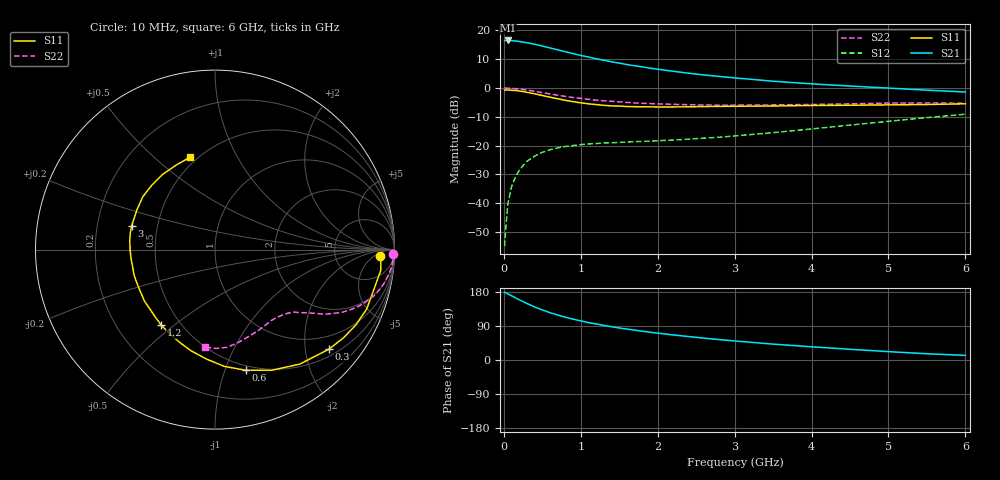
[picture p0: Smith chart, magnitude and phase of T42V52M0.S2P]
! Infineon Technologies  Discrete & RF Semiconductors
! BFR182T
! Si NPN RF Bipolar Junction Transistor in SC75
! VCE = 2.5 V  IC = 2 mA
! Common Emitter S-Parameters:  October  1999
# GHz  S  MA  R  50
!  f  S11  S21  S12  S22
! GHz  MAG  ANG  MAG  ANG  MAG  ANG  MAG  ANG
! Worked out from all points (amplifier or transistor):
!   36 points, 10 MHz to 6 GHz, reference 50 ohm
!   highest |S21| = 16.5 dB at 50 MHz (marker M1)
!   |S21| within 3 dB of that: start of sweep to 660.8 MHz
!   unconditionally stable (mu >= 1): 1.966 GHz to 4.331 GHz
!   at 250 MHz: K = 0.14, MSG = 21.5 dB, |S12| = -26.9 dB
!   at 1.4 GHz: K = 0.78, MSG = 14.0 dB, |S12| = -19.0 dB
!   at 6 GHz: K = 0.83, MSG = 3.9 dB, |S12| = -9.1 dB
!   lowest NFmin = 1.10 dB at 450 MHz
!   S11 on the Smith chart (normalised r, x): 10 MHz: 19, -9; 300 MHz: 0.66, -2.52; 600 MHz: 0.46, -1.18; 1.2 GHz: 0.39, -0.45; 3 GHz: 0.35, +0.12; 6 GHz: 0.46, +0.66
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0.01  0.9177 -2.4  6.671 178.4  0.0018 91.8  0.9899 -1.4
0.02  0.9257 -1.5  6.648 178.2  0.0029 92.8  0.9999 -1.2
0.05  0.9306 -7.2  6.704 174.7  0.0094 87.1  0.9939 -3.0
0.1  0.9132 -13.8  6.62 169.7  0.0194 80.7  0.988 -5.9
0.15  0.9077 -21.4  6.561 164.2  0.0284 77.4  0.9743 -8.7
0.25  0.8686 -34.4  6.297 154.1  0.045 71.1  0.9421 -13.8
0.3  0.8433 -41.1  6.118 149.2  0.0535 68.1  0.9233 -16.1
0.4  0.7937 -53.5  5.767 140.0  0.0659 61.9  0.8772 -20.3
0.5  0.7429 -64.8  5.357 132.2  0.0767 56.7  0.8321 -23.5
0.6  0.6937 -75.7  4.97 124.9  0.0848 52.7  0.7906 -26.2
0.8  0.6124 -94.3  4.275 112.9  0.0967 46.5  0.7162 -30.1
0.9  0.58 -103.1  3.958 107.8  0.1005 44.7  0.6849 -31.5
1.1  0.5326 -118.5  3.451 98.7  0.107 42.0  0.6375 -33.7
1.2  0.517 -125.3  3.225 95.1  0.1088 41.0  0.6171 -34.8
1.4  0.4908 -137.9  2.857 87.9  0.1125 40.0  0.5887 -36.7
1.6  0.4779 -149.8  2.561 81.5  0.1156 40.2  0.5629 -38.2
2.2  0.4703 -174.1  1.958 66.2  0.1254 43.9  0.5223 -44.4
3  0.483 163.9  1.501 50.3  0.1475 51.2  0.5052 -54.0
3.5  0.4882 152.9  1.315 41.9  0.1683 55.2  0.5105 -61.0
4.5  0.5026 134.7  1.084 28.3  0.2277 58.6  0.5323 -75.4
5.5  0.5183 114.7  0.92 16.5  0.3069 56.6  0.5508 -89.4
6  0.5326 105.2  0.854 12.2  0.3512 53.6  0.5452 -95.7
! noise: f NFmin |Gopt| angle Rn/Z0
0.45  1.1  0.42  29  0.36
0.9  1.2  0.4  58  0.3
1.8  1.85  0.32  126  0.22
